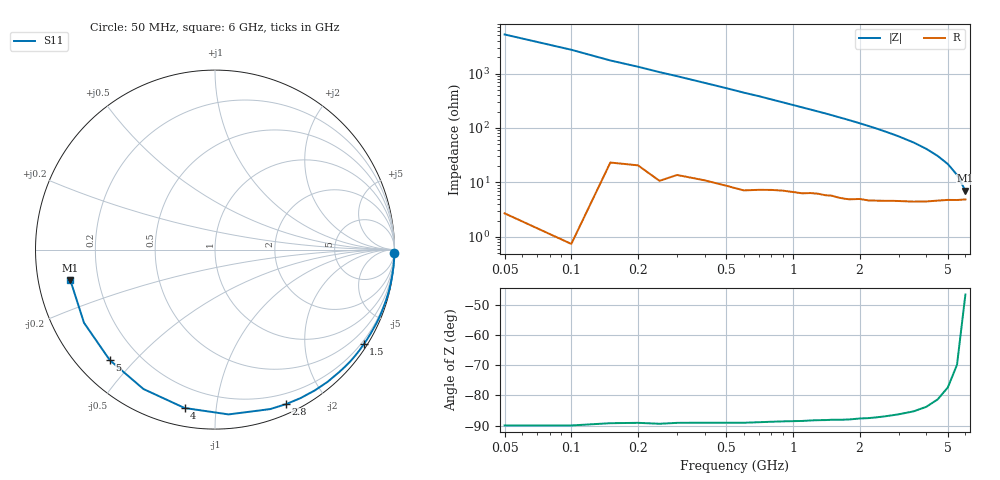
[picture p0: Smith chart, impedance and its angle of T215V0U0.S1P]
! SIEMENS Discrete & RF Semiconductors
! BAS70-04W
! Si Schottky Diode in SOT323
! VR = 15 V
! S-Parameters:  November  1997
# GHz  S  MA  R  50
!  f  S11
! GHz  MAG  ANG
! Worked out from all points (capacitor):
!   34 points, 50 MHz to 6 GHz, reference 50 ohm
!   read as one part to ground: C = 611 fF near 50 MHz
!   lowest |Z| = 7.07 ohm at 6 GHz (marker M1)
!   S11 on the Smith chart (normalised r, x): 50 MHz: open; 1.5 GHz: 0.11, -3.43; 2.8 GHz: 0.09, -1.55; 4 GHz: 0.09, -0.82; 5 GHz: 0.10, -0.43; 6 GHz: 0.10, -0.10
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0.05  1 -1.1
0.1  1 -2.1
0.15  0.9992 -3.3
0.25  0.999 -5.4
0.4  0.9976 -8.5
0.6  0.9964 -12.8
0.7  0.9951 -14.8
0.8  0.9936 -17.0
1  0.9908 -21.4
1.1  0.9895 -23.6
1.4  0.9843 -30.2
1.5  0.9822 -32.5
1.6  0.9811 -34.9
1.7  0.9796 -37.2
1.8  0.9777 -39.6
1.9  0.9749 -42.0
2  0.9718 -44.5
2.2  0.9677 -49.5
2.4  0.9617 -54.6
2.6  0.9549 -60.0
2.8  0.9475 -65.4
3  0.9403 -70.9
3.5  0.9214 -85.3
4  0.8986 -100.9
4.5  0.873 -117.2
5  0.8502 -133.6
5.5  0.836 -150.8
6  0.824 -168.2
